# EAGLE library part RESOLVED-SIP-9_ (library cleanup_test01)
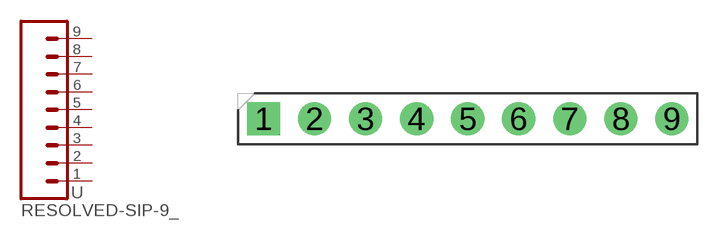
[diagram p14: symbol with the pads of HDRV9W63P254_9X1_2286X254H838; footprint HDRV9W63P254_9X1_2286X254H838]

Designator prefix -

## RESOLVED-SIP-9_2.54-SPACE-VERTICAL  [HDRV9W63P254_9X1_2286X254H838]
1  1  pas
2  2  pas
3  3  pas
4  4  pas
5  5  pas
6  6  pas
7  7  pas
8  8  pas
9  9  pas

## Footprint HDRV9W63P254_9X1_2286X254H838 (pad centres in mm)
drill 1.1 pad 1.65 square: 1 0,0
drill 1.1 pad 1.65: 2 2.54,0; 3 5.08,0; 4 7.62,0; 5 10.16,0; 6 12.7,0; 7 15.24,0; 8 17.78,0; 9 20.32,0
